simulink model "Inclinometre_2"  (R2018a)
settings: Solver=FixedStepAuto  StartTime=0.0  StopTime=inf  RelTol=1e-3  EnableMultiTasking=on
libraries: arduinolib x1

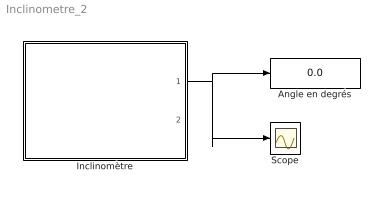
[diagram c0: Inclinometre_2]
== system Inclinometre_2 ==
  Angle en degrés : Display
  Inclinomètre : Subsystem
  Scope : Scope
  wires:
  Inclinomètre/1(d) -> Scope/1, Angle en degrés/1

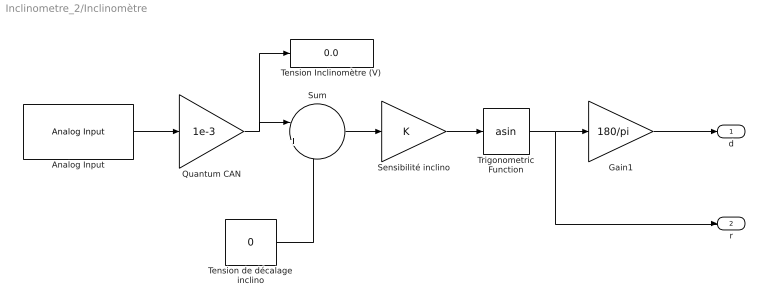
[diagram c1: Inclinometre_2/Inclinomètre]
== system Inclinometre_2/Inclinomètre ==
  Analog Input : arduinolib/Analog Input  pinNumber=4  ReadResultsOnly=off  ConversionTriggerSource=Software  ExternalTriggerType=uint32(0)  OutputDataType=uint16  EnableConversionCompleteNotify=off  EnableOuputStatus=off  SampleTime=0.01  blockPlatform=arduino
  Gain1 : Gain  Gain=180/pi
  Quantum CAN : Gain  Gain=1e-3
  Sensibilité inclino : Gain
  Sum : Sum  Inputs=|+-
  Tension Inclinomètre (V) : Display
  Tension de décalage inclino : Constant  Value=0
  Trigonometric Function : Trigonometry  Operator=asin
  d : Outport
  r : Outport  Port=2
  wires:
  Sensibilité inclino/1 -> Trigonometric Function/1
  Gain1/1 -> d/1
  Trigonometric Function/1 -> r/1, Gain1/1
  Analog Input/1 -> Quantum CAN/1
  Tension de décalage inclino/1 -> Sum/2
  Quantum CAN/1 -> Tension Inclinomètre (V)/1, Sum/1
  Sum/1 -> Sensibilité inclino/1
